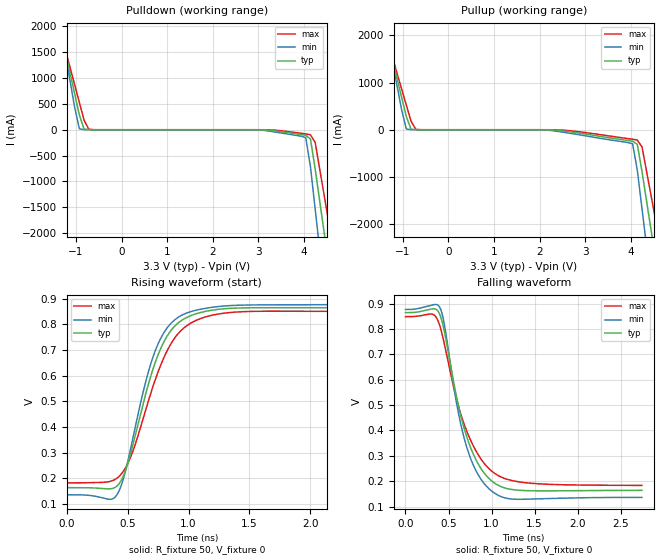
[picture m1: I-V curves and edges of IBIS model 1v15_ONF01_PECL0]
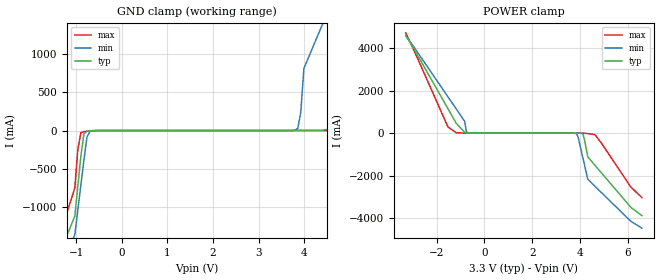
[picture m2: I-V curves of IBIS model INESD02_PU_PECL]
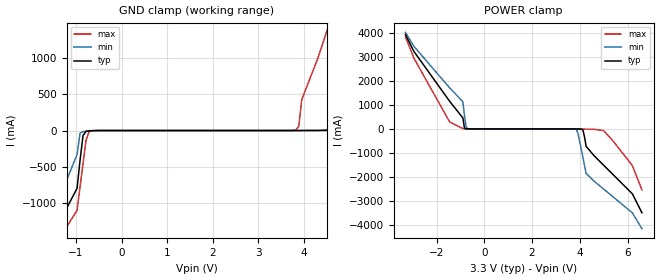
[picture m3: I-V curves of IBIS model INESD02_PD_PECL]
|   This file is an IBIS representation of the   |
|   Integrated Device Technology , Inc.   |
|   ICS85211BI-03   |
|   LOW SKEW, 1-TO-2 DIFFERENTIAL-TO-LVHSTL FANOUT BUFFER   |
[IBIS Ver]   4.1
[File name]   85211bi_03_3v3.ibs
[File Rev]   1.0
[Date]   16 Oct 2009 | Last modified
|   Apr 31 2004 | Generated
[Source]   Originated at Integrated Device Technology, Inc.
[Disclaimer]
IDT hereby grants the user of this IBIS model a non-exclusive,
nontransferable license to use this IBIS model under the following terms.
Before using this IBIS model, the user should read this license.
If the user does not accept these terms,  the IBIS model should be
returned to IDT within 30 days.
   The user is granted this license only to use the IBIS model and
is not granted rights to sell, load, rent, lease or license the IBIS
model in whole or in part, or in modified form to anyone other than
user. User may modify the IBIS model to suit its specific
applications but rights to derivative works and such modifications
shall belong to IDT.
   This IBIS model is provided on an "AS IS" basis and IDT makes
absolutely no warranty with respect to the information contained
herein. IDT DISCLAIMS AND CUSTOMER WAIVES ALL WARRANTIES, EXPRESS
OR IMPLIED, INCLUDING WARRANTIES OF MERCHANTABILITY OR FITNESS FOR
A PARTICULAR PURPOSE. The entire risk as to quality and performance
is with the Customer. ACCORDINGLY, IN NO EVENT SHALL THE COMPANY BE
LIABLE FOR ANY DAMAGES, WHETHER IN CONTRACT OR TORT,INCLUDING ANY
LOST PROFITS OR OTHER INCIDENTAL, CONSEQUENTIAL, EXEMPLARY, OR
PUNITIVE DAMAGES ARISING OUT OF THE USE OR APPLICATION OF THE IBIS
model provided in this package. Further, IDT reserves the right to
make changes without notice to any product herein to improve
reliability, function, or design. IDT does not convey any license
under patent rights or any other intellectual property rights,
including those of third parties.
   IDT is not obligated to provide maintenance or support
for the licensed IBIS model.
[Copyright]   Copyright 2004 by Integrated Device Technology , Inc.
[Component]   ICS85211BMI-03
[Manufacturer] Integrated Device Technology, Inc.
[Package]
|SOIC 8 Lead
|   typ   min   max
R_pkg   57.05m   55.5m   58.6m
L_pkg   1.769nH   1.570nH   1.968nH
C_pkg   0.269pF   0.252pF   0.286pF
[Pin] signal_name   model_name   R_pin   L_pin   C_pin
1   Q0   1v15_ONF01_PECL0   58.6m   1.968n   0.286p
2   nQ0   1v15_ONF01_PECL0   55.5m   1.570n   0.252p
3   Q1   1v15_ONF01_PECL0   55.5m   1.570n   0.252p
4   nQ1   1v15_ONF01_PECL0   56.6m   1.968n   0.286p
5   GND   GND   58.6m   1.968n   0.286p
6   nCLK   INESD02_PU_PECL   55.5m   1.570n   0.252p
7   CLK   INESD02_PD_PECL   55.5m   1.570n   0.252p
8   VDD   POWER   56.6m   1.968n   0.286p
[Diff Pin]  inv_pin  vdiff tdelay_typ tdelay_min  tdelay_max
1   2   NA   0  0  0
3   4   NA   0  0  0
| Models and submodels in the file (3): 1v15_ONF01_PECL0 (Output_ECL), INESD02_PU_PECL (Input), INESD02_PD_PECL (Input)
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[Model]   1v15_ONF01_PECL0
Model_type   Output_ECL
Polarity   Non-Inverting
|   typ   min   max
C_comp   2pF   1.5pF   2.5pF
Vmeas = 0.48V
Rref = 50
Cref = 0
Vref = 0V
|   typ   min   max
[Voltage range]   3.3V   3.135V   3.465V
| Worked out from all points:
|   rising waveform, R_fixture 50, V_fixture 0: 20-80 % time 261ps typ, 245ps min, 295ps max; typ from 0.164 V to 0.865 V
|   falling waveform, R_fixture 50, V_fixture 0: 20-80 % time 302ps typ, 269ps min, 356ps max; typ from 0.865 V to 0.164 V
[Pulldown]
|Voltage   I (typ)   I (min)   I (max)
-3.3V     9.786A     12.03A     8.45A
-1.337V   1.928A     2.007A     1.897A
-923.3mV  281.9mA    16.92mA    525.2mA
-716.7mV  863uA      101.6uA    9.444mA
4.037V    -108.9mA   -151.3mA   -80.62mA
4.14V     -176.2mA   -712.1mA   -97.9mA
4.243V    -757.1mA   -1.533A    -243.9mA
4.347V    -1.402A    -2.354A    -780.4mA
4.45V     -2.046A    -3.176A    -1.318A
4.553V    -2.691A    -3.997A    -1.856A
4.657V    -3.336A    -4.819A    -2.395A
6.6V      -15.7A     -20.58A    -12.71A
[Pullup]
|Voltage   I (typ)   I (min)   I (max)
-3.3V     9.786A     12.03A     8.45A
-1.44V    2.34A      2.533A     2.241A
-1.337V   1.928A     2.007A     1.897A
-923.3mV  281.9mA    16.92mA    525.2mA
-716.7mV  863uA      101.6uA    9.444mA
4.037V    -242.6mA   -297.3mA   -201.2mA
4.14V     -310.1mA   -857.8mA   -219.3mA
4.243V    -891mA     -1.678A    -365.9mA
4.347V    -1.535A    -2.499A    -902.6mA
4.45V     -2.18A     -3.32A     -1.441A
4.657V    -3.468A    -4.961A    -2.517A
6.6V      -15.69A    -20.54A    -12.72A
[Ramp]
|   typ   min   max
dV/dt_r   0.564/0.407n   0.607/0.388n   0.534/0.466n
dV/dt_f   0.574/0.469n   0.614/0.431n   0.541/0.548n
R_load =   50.0000
[Rising Waveform]
R_fixture = 50
V_fixture = 0
V_fixture_max = 0
V_fixture_min = 0
C_fixture = 0.0p
| Time   typ   min   max
0s        163.7mV    136mV      182.4mV
412.9ps   170.4mV    136.7mV    200.9mV
465.2ps   209.9mV    199mV      228.1mV
531.3ps   308.9mV    330.4mV    290.9mV
633.1ps   502.2mV    548.1mV    442.7mV
713ps     632.5mV    679.4mV    565.3mV
814.8ps   746.9mV    779.9mV    688mV
933.2ps   812.1mV    832.6mV    773.2mV
1.346ns   862.3mV    873.1mV    846.2mV
2.747ns   864.8mV    877.2mV    849.6mV
[Falling Waveform]
R_fixture = 50
V_fixture = 0
V_fixture_max = 0
V_fixture_min = 0
C_fixture = 0.0p
| Time   typ   min   max
0s        864.9mV    877.3mV    849.1mV
313.8ps   880.1mV    895.6mV    858.6mV
401.9ps   854.8mV    883.3mV    809.8mV
457ps     782.9mV    808.6mV    733.3mV
602.9ps   516.6mV    490.1mV    511.3mV
693.7ps   394.6mV    355mV      413.5mV
828.6ps   278mV      235mV      313.6mV
1.002ns   200.8mV    160.7mV    239.6mV
1.429ns   162.4mV    129mV      192.6mV
2.747ns   163.7mV    136mV      183.2mV
[Model]   INESD02_PU_PECL
Model_type  Input
Polarity   Non-Inverting
Vinl = 0.8V
Vinh = 2.0V
|   typ   min   max
C_comp   2pF   1.5pF   2.5pF
|   typ   min   max
[Voltage range]  3.3V   3.15V   3.45V
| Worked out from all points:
|   GND clamp passes 1 mA (typ) near -0.59 V on its own axis
|   POWER clamp passes 1 mA (typ) near -0.70 V on its own axis
[GND_clamp]
|Voltage   I(typ)   I(min)   I(max)
-3.3V     -3.894A    -3.674A    -4.294A
-1.3V     -1.521A    -1.7A      -1.261A
-1.031V   -1.125A    -1.372A    -755.3mA
-896.9mV  -335.4mA   -714.7mA   -27.07mA
-695.9mV  -3.401mA   -10.69mA   -6.477mA
3.794V    17.99uA    3.319mA    6.081uA
3.928V    181.1uA    239mA      10.12uA
3.995V    711.6uA    813.7mA    20.78uA
4.8V      40.44mA    1.967A     268.6uA
5.6V      1.139A     3.12A      2.243mA
6.3V      2.525A     4.275A     64.01mA
6.6V      3.219A     4.852A     752.7mA
[POWER_clamp]
|Voltage   I(typ)   I(min)   I(max)
-3.3V     4.617A     4.594A     4.726A
-1.53V    1.149A     1.709A     289.6mA
-1.18V    456.4mA    1.132A     15.33mA
-829.9mV  42.02mA    556.1mA    3.39mA
-762.9mV  4.159mA    91mA       1.422mA
-695.9mV  727.9uA    10.66mA    491.6uA
3.861V    -620.9uA   -26.2mA    -103.4uA
4.129V    -41.91mA   -1.19A     -4.968mA
4.33V     -1.119A    -2.176A    -17.93mA
4.63V     -1.515A    -2.505A    -71.45mA
6.13V     -3.492A    -4.151A    -2.536A
6.6V      -3.888A    -4.48A     -3.041A
[Model]   INESD02_PD_PECL
Model_type  Input
Polarity   Non-Inverting
Vinl = 0.8V
Vinh = 2.0V
|   typ   min   max
C_comp   2pF   1.5pF   2.5pF
|   typ   min   max
[Voltage range]  3.3V   3.15V   3.45V
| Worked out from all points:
|   GND clamp passes 1 mA (typ) near -0.59 V on its own axis
|   POWER clamp passes 1 mA (typ) near -0.70 V on its own axis
[GND_clamp]
-3.3V     -3.894A    -4.294A    -3.674A
-1.6V     -1.569A    -1.322A    -1.74A
-974.8mV  -794.1mA   -331.5mA   -1.096A
-843.4mV  -68.33mA   -15.34mA   -452.9mA
-646.5mV  -1.912mA   -4.151mA   -2.665mA
3.818V    89.38uA    70.49uA    7.198mA
3.95V     342.2uA    75.94uA    423.8mA
4.6V      7.437mA    165.5uA    1.553A
4.9V      78.32mA    440.9uA    2.118A
5.5V      1.293A     2.769mA    3.249A
6.25V     2.651A     112.4mA    4.38A
6.6V      3.331A     896.1mA    4.946A
[POWER_clamp]
-3.3V     3.923A     4.017A     3.838A
-2.95V    3.23A      3.44A      2.951A
-1.45V    1.149A     1.709A     289.6mA
-896.9mV  456.5mA    1.133A     15.4mA
-762.9mV  4.223mA    91.07mA    1.486mA
-695.9mV  792.2uA    10.73mA    555.6uA
3.861V    -556.7uA   -26.14mA   -39.45uA
4.129V    -41.85mA   -1.19A     -4.904mA
4.263V    -724.2mA   -1.847A    -12.04mA
5V        -1.514A    -2.505A    -71.38mA
6.2V      -2.701A    -3.492A    -1.525A
6.6V      -3.492A    -4.151A    -2.536A
